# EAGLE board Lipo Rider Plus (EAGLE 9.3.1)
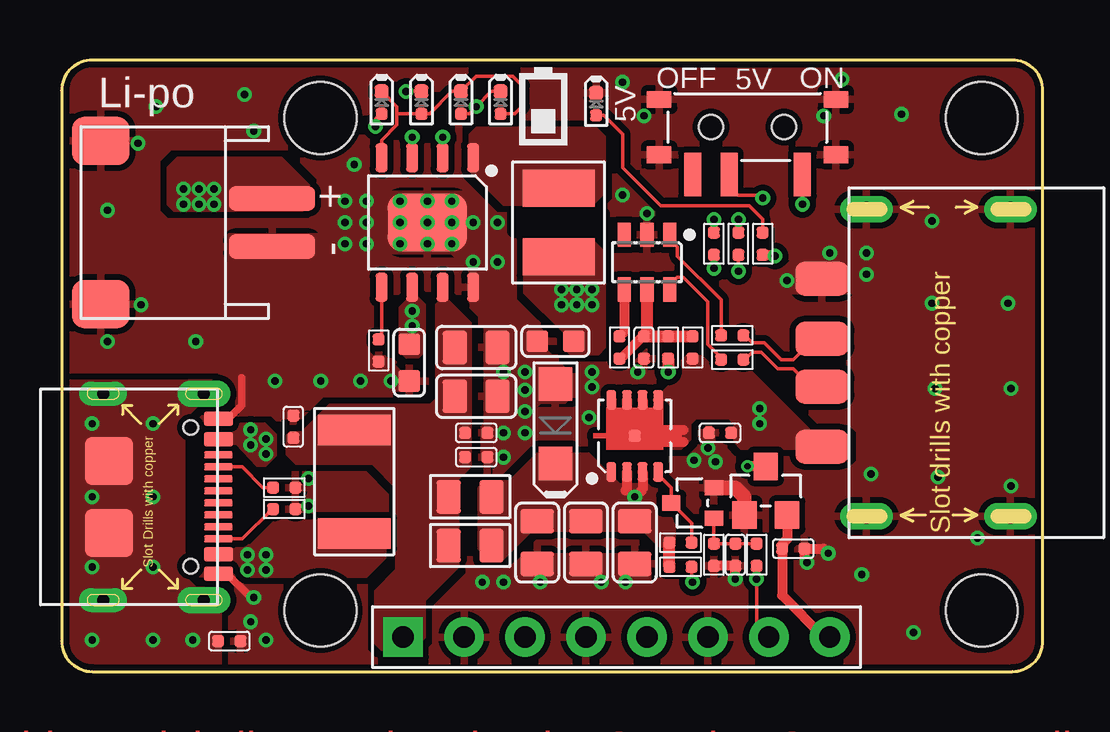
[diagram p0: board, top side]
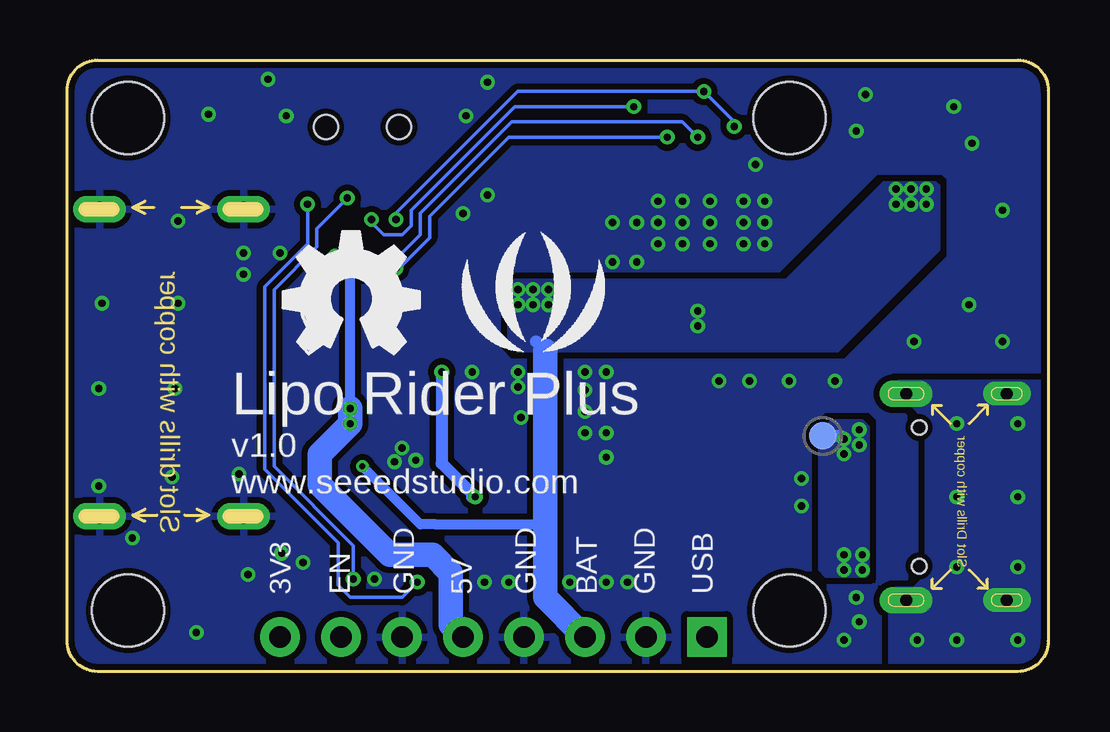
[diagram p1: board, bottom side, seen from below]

Size 40.88 x 25.48 mm. Coordinates in mm from the lower left corner, seen from the top.
Outline: 0,24.21 0,1.27 arc90 1.27,0 39.61,0 arc90 40.88,1.27 40.88,24.21 arc90 39.61,25.48 1.27,25.48 arc90 0,24.21
Copper layers (1*16): Top 0.035mm / dielectric 1.5mm / Bottom 0.035mm
Design rules "SeeedStudio_2layer_DRU_no_angle_20140221 *": minimum track width 1mil, minimum drill 10mil, track to track 6mil, track to pad 6mil, pad to pad 6mil, via to via 6mil, smd to smd 0mil, copper to edge 10mil, drill to drill 10mil, minimum pad ring 4mil, minimum via ring 4mil, stop-mask expansion 2mil, vias tented up to drill 25mil, thermal gap 10mil
Holes 3 mm at 10.78,23.07 10.78,2.54 38.34,23.07 38.34,2.54
tRestrict: area 18.8,18.3 to 22.6,19.1

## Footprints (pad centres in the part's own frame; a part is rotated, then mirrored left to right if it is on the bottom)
C0402 = smd 0.5 x 0.5: 1 -0.463,0; 2 0.463,0
C0603 = smd 0.889 x 0.889: 1 -0.762,0; 2 0.762,0
C0805 = smd 1.016 x 1.397: 1 -0.889,0; 2 0.889,0
ESD-0402 = smd 0.5 x 0.5: 1 -0.463,0; 2 0.463,0
LED-0402 = smd 0.5 x 0.5: + 0.463,0 | smd 0.58 x 0.58: - -0.468,0
SOD-123 = smd 1.397 x 1.397: + 1.651,0; - -1.651,0
F1812 = smd 1.27 x 3.048: 1 -2.159,0; 2 2.159,0
F0805 = smd 1.016 x 1.397: 1 -0.889,0; 2 0.889,0
USB4+4P-2.0-14.6X10.6X5.72MM = smd 1.4 x 2.2: 1 -3.5,0.5; 2 -1,0.5; 3 1,0.5; 4 3.5,0.5 | drill 0.6 pad 1.1 long: S1 -6.4,-1.35; S2 6.4,-1.35; S3 -6.4,-7.35; S4 6.4,-7.35
H8-2.54-C65D35MIL = drill 0.889 pad 1.651 square: 1 0,8.89 | drill 0.889 pad 1.651: 2 0,6.35; 3 0,3.81; 4 0,1.27; 5 0,-1.27; 6 0,-3.81; 7 0,-6.35; 8 0,-8.89
HW2-SMD-2.0-90D = smd 2 x 2.4: 3 3.4,-2.181; 4 -3.4,-2.181 | smd 1 x 3.6: + -1,4.953; - 1,4.953
L4.4X3.0MM = smd 1.55 x 3: 1 -1.425,0; 2 1.425,0
DFN8P-0.65-3X3X0.8MM = smd 0.8 x 0.4: 1 -1.5,0.975; 2 -1.5,0.325; 3 -1.5,-0.325; 4 -1.5,-0.975; 5 1.5,-0.975; 6 1.5,-0.325; 7 1.5,0.325; 8 1.5,0.975 | smd 0.508 x 0.508: 9 0,0
SOT-323 = smd 0.762 x 0.635: 1 0.889,-0.635; 2 0.889,0.635; 3 -0.889,0
R0402 = smd 0.5 x 0.5: 1 -0.463,0; 2 0.463,0
SW7-SMD-L6.7X2.7X3.2MM = smd 1.8 x 0.7: 1 1.978,2.286; 2 1.978,-0.762; 3 1.978,-2.286 | smd 0.7 x 1.016: SS1 -1.15,-3.683; SS2 1.15,-3.683; SS3 1.15,3.683; SS4 -1.15,3.683 | hole 1: 0,-1.524; 0,1.524
TP-D45MIL = smd 1.143 x 1.143: T 0,0
ESOP8L-1.27-5X3.9MM = smd 0.5 x 1.2: 1 -1.905,-2.7; 2 -0.635,-2.7; 3 0.635,-2.7; 4 1.905,-2.7; 5 1.905,2.7; 6 0.635,2.7; 7 -0.635,2.7; 8 -1.905,2.7 | smd 3.3 x 2.4: PAD 0,0
SOT-23-6 = smd 0.55 x 1.016: 1 -0.95,-1.143; 2 0,-1.143; 3 0.95,-1.143; 4 0.95,1.143; 5 0,1.143; 6 -0.95,1.143
SOT-23 = smd 1.016 x 1.143: 1 -0.889,-1.016; 2 0.889,-1.016; 3 0,1.016
USB2.0-TYPE-C = smd 1.2 x 0.6: A1_B12 0.05,3.25; A4_B9 0.05,2.4; B1_A12 0.05,-3.2; B4_A9 0.05,-2.4 | smd 1.2 x 0.3: A5 0.05,1.25; A6 0.05,0.25; A7 0.05,-0.25; A8 0.05,-1.25; B5 0.05,-1.75; B6 0.05,-0.75; B7 0.05,0.75; B8 0.05,1.75 | drill 0.5 pad 1 long: S1 -4.75,4.3; S2 -4.75,-4.3 | drill 0.5 pad 1.1 long: S3 -0.55,4.3; S4 -0.55,-4.3 | smd 2 x 2: S5 -4.5,1.5; S6 -4.5,-1.5 | hole 0.6: -1.1,-2.89; -1.1,2.89

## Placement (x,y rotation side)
C1  100nF  [C0402]  17.27,8.93 0 top
C2  100nF  [C0402]  17.27,9.95 0 top
C3  10uF  [C0603]  14.48,12.87 270 top
C4  10uF  [C0603]  20.57,13.76 180 top
C5  10uF/10V  [C0805]  17.27,11.47 180 top
C6  10uF/10V  [C0805]  17.27,13.5 180 top
C7  10uF/10V  [C0805]  21.84,5.37 90 top
C8  10uF/10V  [C0805]  19.81,5.37 90 top
C9  10uF/10V  [C0805]  23.88,5.37 90 top
C12  100nF  [C0402]  30.48,5.12 0 top
C13  100nF  [C0402]  24.26,13.5 270 top
C42  10nF  [C0402]  28.07,4.87 270 top
C43  100nF  [C0402]  27.43,9.95 180 top
D1  ESDPSA0402V05  [ESD-0402]  9.65,10.2 270 top
D2  GREEN  [LED-0402]  13.34,23.7 270 top
D3  GREEN  [LED-0402]  14.99,23.7 270 top
D4  GREEN  [LED-0402]  18.29,23.7 270 top
D5  GREEN  [LED-0402]  16.64,23.7 270 top
D6  MMSZ4689-E3-08  [SOD-123]  20.57,10.33 90 top
D7  GREEN  [LED-0402]  22.27,23.64 270 top
F1  3A  [F1812]  12.19,7.91 90 top
FB1  1.5A  [F0805]  17.02,5.25 0 top
FB2  1.5A  [F0805]  17.02,7.28 0 top
FR1  SEEEDSTUDIO-OPEN-SCH-FRAME-BIG  [SEEEDSTUDIO-PCB-FRAME]  not placed on the board
FR2  SEEEDSTUDIO-OPEN-SCH-FRAME-BIG  [SEEEDSTUDIO-PCB-FRAME]  not placed on the board
J2  [USB4+4P-2.0-14.6X10.6X5.72MM]  32.18,12.87 90 top
J3  [H8-2.54-C65D35MIL]  23.11,1.44 90 top
J4  320110026  [HW2-SMD-2.0-90D]  3.81,18.71 270 top
L1  1uF  [L4.4X3.0MM]  20.7,18.71 90 top
Q1  AON7403  [DFN8P-0.65-3X3X0.8MM]  23.88,9.82 90 top
Q2  2N7002PW  [SOT-323]  26.29,7.03 0 top
R1  56k  [R0402]  13.21,13.38 90 top
R2  1k  [R0402]  27.18,17.82 90 top
R3  1k  [R0402]  29.21,17.82 270 top
R4  DNP  [R0402]  25.27,13.5 270 top
R5  0R  [R0402]  23.24,13.5 270 top
R6  22R  [R0402]  27.94,12.99 0 top
R7  5.1k  [R0402]  9.27,7.66 180 top
R8  5.1k  [R0402]  9.27,6.77 0 top
R9  1k  [R0402]  28.19,17.82 90 top
R10  22R  [R0402]  27.94,14.01 0 top
R11  2.2k  [R0402]  26.29,13.5 270 top
R12  0R  [C0402]  6.99,1.27 0 top
R32  100k  [R0402]  25.78,5.37 0 top
R46  100k  [R0402]  27.18,4.87 90 top
R47  10k  [R0402]  25.78,4.36 180 top
R48  1k  [R0402]  28.96,4.87 90 top
SW1  311030001  [SW7-SMD-L6.7X2.7X3.2MM]  28.57,22.69 270 top
TP1  TEST  [TP-D45MIL]  9.4,9.82 0 bottom
U1  ETA9740  [ESOP8L-1.27-5X3.9MM]  15.24,18.71 180 top
U2  [SOT-23-6]  24.38,17.06 180 top
U3  [SOT-23]  29.34,7.53 0 top
U$1  [SEEED-SILK-TNAME-280*268MIL]  21.46,15.03 0 bottom
U$2  [OSHW_FILLX200_NOTEXT_TNAME]  31.88,13.25 0 bottom
USB2  TYPE-C  [USB2.0-TYPE-C]  6.48,7.28 0 top

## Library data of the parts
C1-C9 C12 C13 C42 C43 D1-D7 F1 FB1 FB2 L1 Q1 Q2 R1-R12 R32 R46-R48 SW1 = Discrete-new
FR1 FR2 = moudle-new
J2-J4 USB2 = Connector-new
TP1 = Discrete-new; PARTNO: DNP
U1-U3 = IC-new
U$1 U$2 = logo

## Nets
3V3: C12.1 J3.8 U3.2
5V: C43.1 J2.1 J3.5 Q1.5 Q1.6 Q1.7 Q1.8 Q1.9 R3.2 R11.2
BAT: C3.1 C4.1 J3.3 J4.+ L1.1 U1.6 U3.3
D+: J2.3 R10.2
D-: J2.2 R6.2
EN: J3.7 R48.1 SW1.2
GND: C1.2 C2.2 C3.2 C4.2 C5.1 C6.1 C7.1 C8.1 C9.1 C12.2 C13.2 C42.2 C43.2 D1.1 D6.+ D7.- J2.4 J2.S1 J2.S2 J2.S3 J2.S4 J3.2 J3.4 J3.6 J4.3 J4.4 J4.- Q2.2 R1.1 R7.1 R8.2 R12.2 R46.1 SW1.SS1 SW1.SS2 SW1.SS3 SW1.SS4 U1.8 U1.PAD U2.2 U3.1 USB2.A1_B12 USB2.B1_A12
LED1: D2.+ D3.- R2.2
LED2: D4.- D5.+ R9.2
LED3: D2.- D3.+ D4.+ D5.- U1.4
N$1: R7.2 USB2.A5
N$2: R8.1 USB2.B5
N$3: R47.1 SW1.1
N$4: F1.1 TP1.T USB2.A4_B9 USB2.B4_A9
N$6: D7.+ R3.1
N$7: R1.2 U1.5
N$8: L1.2 U1.1
N$9: R9.1 U1.3
N$10: R5.1 U2.4
N$11: C13.1 R4.1 R5.2 R11.1 U2.5
N$12: R2.1 U1.2
N$13: R6.1 U2.6
N$14: R10.1 U2.1
N$49: Q1.4 Q2.3 R32.2
N$52: C42.1 Q2.1 R46.2 R48.2
SHIELD: R12.1 USB2.S1 USB2.S2 USB2.S3 USB2.S4 USB2.S5 USB2.S6
VCC_5V: C7.2 C8.2 C9.2 D6.- FB1.2 FB2.2 Q1.1 Q1.2 Q1.3 R4.2 R32.1 R47.2
VUSB: C1.1 C2.1 C5.2 C6.2 D1.2 F1.2 FB1.1 FB2.1 J3.1 U1.7

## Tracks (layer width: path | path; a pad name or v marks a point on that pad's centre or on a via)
3V3
  Top 0.406: J3.8 31.75,1.44 30.02,3.17 C12.1 30.02,5.29 30.23,5.5 U3.2
5V  (via drill 0.3 pad 0.61)
  Top 0.406: 29.04,11.01 v29.08,10.96 | R3.2 29.67,17.36 v29.72,17.31 | Q1.5 24.85,10.54 24.77,10.45 | Q1.6 24.2,10.64 24.77,10.07 24.89,10.07 | Q1.7 23.55,10.4 23.62,10.33 | Q1.8 22.9,10.41 22.99,10.33 | 24.89,10.07 25.91,10.07 | 24.89,10.07 24.89,9.69 25.02,9.56 25.65,9.56 | 25.65,9.56 25.91,9.56 | 25.65,9.56 25.65,9.95
  Bottom 0.406: v29.08,10.96 29.08,16.68 v29.72,17.31
  Bottom 1.016: v29.08,10.96 v29.08,10.33 30.35,9.06 30.35,7.79 27.43,4.87 25.65,4.87 24.89,4.1 24.89,1.95 J3.5
  pour Top (isolate 0.254, no thermals): 32.51,8.8 31.37,8.8 30.86,9.31 28.32,9.31 28.07,9.56 28.07,10.33 27.81,10.58 26.42,10.58 26.16,10.33 26.16,9.67 25.8,9.31 23.11,9.31 22.73,9.69 22.73,10.58 22.99,10.84 24.64,10.84 24.89,11.09 24.89,11.47 25.78,12.36 25.78,12.87 26.04,13.12 26.67,13.12 27.3,12.49 28.7,12.49 31.24,9.95 32.51,9.95 32.77,9.69 32.77,9.06
BAT  (via drill 0.25 pad 0.51, 0.3 pad 0.61)
  Top 0.406: U3.3 v28.57,8.55
  Bottom 0.406: 20.95,6.26 21.08,6.14 25.27,6.14 25.53,6.14 26.16,6.14 v28.57,8.55
  Bottom 0.508: 20.95,13.38 C4.1
  Bottom 1.016: 20.95,13.38 20.95,6.26 20.95,3.09 J3.3
  other vias: 22.1,15.28 21.46,15.28 21.46,15.91 22.1,15.91 20.83,15.91 20.83,15.28 6.35,20.11 6.35,19.47 5.71,19.47 5.71,20.11 5.08,20.11 5.08,19.47 14.61,15.03 14.61,14.39
  pour Top (isolate 0.254, no thermals): 10.03,19.22 4.7,19.22 4.45,19.47 4.45,21 4.83,21.38 9.14,21.38 10.29,20.23 10.29,19.47
  pour Top (isolate 0.254, no thermals): 14.61,16.3 14.48,16.17 14.48,15.53 14.1,15.15 14.1,13.38 14.35,13.12 14.86,13.12 15.11,13.38 15.11,15.28 14.86,15.53 14.73,15.66 14.73,16.17
  pour Top (isolate 0.254, no thermals): 22.1,13.25 21.21,13.25 20.95,13.5 20.95,14.14 19.3,15.79 19.3,17.69 19.56,17.95 22.1,17.95 22.61,17.44 22.61,13.5 22.35,13.25
  pour Bottom (isolate 0.254, no thermals): 21.84,16.3 10.92,16.3 6.86,20.36 4.7,20.36 4.57,20.23 4.57,17.57 8.76,13.38 22.1,13.38 22.48,13.76 22.48,16.04 22.23,16.3
D+
  Top 0.152: R10.2 28.45,14.01 28.77,13.69 29.27,13.69 29.97,12.99 30.48,12.99 31.35,13.87 J2.3
D-
  Top 0.152: R6.2 28.45,12.99 28.77,13.31 29.15,13.31 29.84,12.61 30.48,12.61 31.18,11.91 31.23,11.87 J2.2
EN  (via drill 0.3 pad 0.61)
  Top 0.152: 28.96,4.49 R48.1 v28.96,3.85 28.96,1.95 J3.7 | v29.21,19.73 29.08,19.85 28.19,19.85 27.81,20.23 SW1.2
  Bottom 0.152: v28.96,3.85 28.96,5.25 32.26,8.55 32.26,15.91 30.48,17.69 30.48,18.45 v29.21,19.73
GND  (via drill 0.3 pad 0.61)
  Top 0.305: USB2.B1_A12 6.88,4.08 7.75,3.21 | USB2.A1_B12 6.93,10.53 7.49,11.09 7.49,12.23
  Top 0.406: R46.1 C42.2 v28.07,3.85 | v31.05,4.55 30.94,4.66 C12.2 31.75,5.12 v31.94,4.93
  Top 0.61: Q2.2 28.07,7.66 28.45,7.28 U3.1
  other vias: 18.41,9.95 18.41,8.93 19.3,9.95 19.3,10.84 19.3,11.72 19.3,12.49 18.41,12.49 15.24,18.71 15.24,19.6 15.24,17.82 14.1,17.82 14.1,18.71 14.1,19.6 16.26,19.6 16.26,18.71 16.26,17.82 17.14,17.06 18.16,17.06 18.16,18.71 17.14,18.71 12.7,19.6 12.7,18.71 12.7,17.82 11.81,17.82 11.81,18.71 11.81,19.6 13.72,12.11 12.45,12.11 10.79,12.11 8.89,12.11 3.3,15.28 3.17,22.01 19.94,3.72 18.41,3.72 17.53,3.72 22.48,3.72 23.5,3.72 24,12.49 26.92,9.31 26.35,8.8 27.24,8.74 24.38,19.09 23.37,24.55 24.26,23.15 32.51,24.68 31.75,23.15 8,3.09 7.87,2.07 8.51,1.31 3.94,23.54 7.62,24.04 1.91,19.22 5.59,13.76 22.1,12.49 32,17.44 33.53,17.44 33.53,16.55 30.23,16.3 23.37,19.85 22.1,11.85 21.97,10.58 1.91,13.76 8,22.52 12.19,21.12 10.29,8.04 10.29,6.9 33.72,8.23 33.34,4.04 38.16,5.56 39.56,7.72 36.51,8.1 36.39,11.79 39.56,11.79 39.43,15.34 36.26,15.34 36.26,18.77 34.99,23.22 35.5,1.63
  pour Top (isolate 0.254, no thermals): 17.65,8.68 18.41,8.68 19.56,9.82 19.56,10.84 19.94,11.22 20.95,11.22 21.21,11.47 22.23,11.47 22.35,11.6 22.35,12.11 22.1,12.36 21.21,12.36 20.19,13.38 20.19,14.01 18.54,15.66 18.54,18.71 18.29,18.96 17.91,18.96 16.89,19.98 11.81,19.98 11.56,19.73 11.56,18.96 10.79,18.2 6.99,18.2 6.99,13.38 8.64,11.72 8.64,10.96 9.02,10.58 9.78,10.58 10.92,11.72 14.48,11.72 14.73,11.98 14.73,12.36 14.61,12.49 14.1,12.49 13.46,13.12 12.97,13.12 12.67,13.42 12.67,16.77 13.34,17.44 16.26,17.44 17.02,16.68 17.02,15.41 17.65,14.77 17.65,10.33 17.53,10.2 17.53,8.8
  pour Top (isolate 0.254, no thermals): 23.75,4.87 24.13,4.87 24.51,4.49 24.51,3.34 24.13,2.96 16.76,2.96 16.51,3.21 16.51,3.6 17.02,4.1 18.54,4.1 19.3,4.87
  pour Top (isolate 0.254, no thermals): 26.8,10.07 26.67,9.95 26.67,9.44 26.16,8.93 26.16,8.55 26.29,8.42 26.42,8.42 26.8,8.04 26.8,7.53 26.92,7.41 27.94,7.41 28.26,7.72 28.26,8.04 27.81,8.8 27.18,9.56 27.18,9.95 27.05,10.07
  pour Top (isolate 0.254, no thermals): 8.38,3.47 8.13,3.47 7.37,2.71 7.37,1.18 7.62,0.93 8.64,0.93 8.89,1.18 8.89,3.09 8.51,3.47
  pour Top (isolate 0.254, no thermals): 32.51,15.79 33.91,15.79 34.29,16.17 34.29,17.44 34.04,17.69 30.99,17.69 29.97,16.68 29.97,16.17 30.23,15.91 30.35,15.79
  pour Top (isolate 0.254, rank 6): -0.64,26.07 41.7,26.07 41.7,-0.59 -0.64,-0.59
  pour Bottom (isolate 0.254, rank 6): -0.64,26.07 41.7,26.07 41.7,-0.59 1.91,-0.59 1.91,-1.23 -0.64,-1.23
  pour Top (isolate 0.254): 31.62,5.63 31.24,5.63 30.73,5.12 30.73,3.47 30.99,3.21 31.24,3.21 31.5,3.47 31.5,3.98 32.13,4.61 32.13,5.25 31.75,5.63
LED1  (via drill 0.3 pad 0.61)
  Top 0.152: D2.+ 13.29,23.24 13.08,23.03 v13.08,22.71 | R2.2 v27.18,18.84 | D3.- v14.35,24.17
  Bottom 0.152: v27.18,18.84 27.18,19.09 22.1,24.17 v14.35,24.17 13.08,22.9 v13.08,22.71
LED2  (via drill 0.3 pad 0.61)
  Top 0.152: R9.2 v28.19,18.84 | D4.- 17.91,24.17 v17.27,23.54 16.98,23.24 D5.+
  Bottom 0.152: v17.27,23.54 22.23,23.54 26.54,19.22 26.54,18.58 26.92,18.2 27.69,18.2 28.19,18.71 v28.19,18.84
LED3
  Top 0.152: U1.4 13.34,22.14 13.97,22.77 13.97,23.28 | 13.97,23.28 13.97,23.54 D2.- | D2.- | 13.97,23.28 14.01,23.24 D3.+ 15.32,23.24 16.26,24.17 D5.- 17.27,24.8 18.8,24.8 19.18,24.42 19.18,23.54 18.88,23.24 D4.+
N$1
  Top 0.152: USB2.A5 7.51,8.53 8.38,7.66 R7.2
N$2
  Top 0.152: USB2.B5 7.52,5.53 8.76,6.77 R8.1
N$3  (via drill 0.3 pad 0.61)
  Top 0.152: R47.1 26.24,3.77 v26.29,3.72 | SW1.1 v30.86,19.47
  Bottom 0.152: v26.29,3.72 26.92,3.09 29.08,3.09 29.59,3.6 29.59,5.37 32.64,8.42 32.64,16.04 30.86,17.82 v30.86,19.47
N$4  (via drill 0.3 pad 0.61)
  Bottom 0.508: TP1.T 8.64,9.82 v8.51,9.69
  other vias: 8.51,9.06 7.87,9.44 7.87,10.07 7.75,4.87 8.51,4.87 8.51,4.23 7.75,4.23
  pour Top (isolate 0.254, no thermals): 6.16,9.82 6.99,9.82 7.47,10.3 8.45,10.3 8.89,9.86 8.89,9.01 8.48,8.59 8.15,8.59 7.3,9.5 6.22,9.5 6.1,9.63 6.1,9.76
  pour Bottom (isolate 0.254, no thermals): 7.87,10.45 7.75,10.45 7.49,10.2 7.49,4.1 7.62,3.98 9.27,3.98 9.53,4.23 9.53,9.95 9.02,10.45
  pour Top (isolate 0.254, no thermals): 6.35,4.99 7.11,4.99 7.37,5.25 7.87,5.25 8.89,6.26 13.21,6.26 13.46,6.01 13.46,4.74 12.7,3.98 7.87,3.98 7.11,4.74 6.35,4.74 6.22,4.87
N$6
  Top 0.152: R3.1 29.21,18.84 28.64,19.41 24.96,19.41 23.37,21 23.37,22.39 22.58,23.18 D7.+
N$7
  Top 0.152: U1.5 13.34,13.96 R1.2
N$8
  pour Top (isolate 0.254, no thermals): 17.02,20.87 17.02,22.36 17.3,22.65 22.25,22.65 22.61,22.29 22.61,19.98 22.1,19.47 18.41,19.47
N$9  (via drill 0.3 pad 0.61)
  Top 0.152: U1.3 v14.61,22.27 | v28.19,16.68 R9.1
  Bottom 0.152: v28.19,16.68 27.43,17.44 26.92,17.44 26.16,18.2 26.16,19.09 22.35,22.9 15.24,22.9 v14.61,22.27
N$10
  Top 0.406: U2.4 23.43,14.16 R5.1
N$11
  Top 0.406: R5.2 23.29,13.04 24.21,13.96 C13.1
  Top 0.508: U2.5 24.38,14.14 24.26,14.01 C13.1 R4.1 R11.1
N$12  (via drill 0.3 pad 0.61)
  Top 0.152: U1.2 v15.88,22.27 | R2.1 v27.18,16.8
  Bottom 0.152: v15.88,22.27 22.48,22.27 25.78,18.96 25.78,18.07 27.05,16.8 v27.18,16.8
N$13
  Top 0.152: R6.1 27.48,13.07 26.92,13.63 26.92,15.41 25.91,16.42 25.65,16.42 25.33,16.1 U2.6
N$14
  Top 0.152: R10.1 27.48,15.49 25.65,17.31 25.65,17.69 25.33,18.01 U2.1
N$49
  Top 0.152: R32.2 26.24,6.18 Q2.3 25.4,7.66 24.85,8.21 Q1.4
N$52
  Top 0.152: R48.2 C42.1 R46.2 Q2.1
SHIELD  (via drill 0.3 pad 0.61)
  other vias: 5.46,1.31 3.81,1.31 1.27,1.31 1.27,4.36 3.81,4.36 3.81,7.28 1.27,7.28 1.27,10.33 3.81,10.33
  pour Top (isolate 0.254, no thermals): 0,12.11 6.22,12.11 6.48,11.85 6.48,11.47 6.22,11.22 5.76,11.22 5.08,10.53 5.08,3.98 5.59,3.47 6.35,3.47 6.6,3.21 6.6,0.04 0,0.04
  pour Bottom (isolate 0.254, no thermals): 0,12.11 6.22,12.11 6.48,11.85 6.48,11.47 6.22,11.22 5.82,11.22 5.08,10.48 5.08,3.99 5.6,3.47 6.35,3.47 6.6,3.21 6.6,0.04 0,0.04
VCC_5V  (via drill 0.3 pad 0.61)
  Top 0.406: Q1.2 23.55,7.59 23.5,7.53 | Q1.3 24.2,7.6 v23.88,7.28
  Top 0.508: R4.2 v25.27,12.49 | R47.2 R32.1
  Bottom 0.508: v25.27,12.49 25.27,8.68 v23.88,7.28 24,7.28
  pour Top (isolate 0.254, no thermals): 17.65,7.91 18.67,7.91 19.81,9.06 21.97,9.06 23.24,7.79 24.64,7.79 25.15,7.03 25.53,6.01 25.53,5.37 25.4,5.25 24.89,5.25 24.26,5.88 19.56,5.88 18.41,4.74 17.78,4.74 17.4,5.12 17.4,7.66
VUSB
  pour Top (isolate 0.254, no thermals): 15.88,16.17 15.75,16.04 15.75,15.41 15.62,15.28 15.62,11.34 15.37,11.09 11.18,11.09 10.03,9.95 9.53,9.95 9.4,9.82 9.4,9.06 9.78,8.68 12.95,8.68 13.97,7.66 13.97,4.23 13.08,3.34 13.08,1.18 13.34,0.93 14.61,0.93 15.11,1.44 15.11,2.96 16.51,4.36 16.51,8.04 17.02,8.55 17.02,14.52 16,15.53 16,16.04

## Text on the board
tNames: OFF | 5V | ON | Li-po | 5V | + | -
bNames: Lipo Rider Plus | v1.0 | www.seeedstudio.com | USB | GND | BAT | GND | 5V | GND | EN | 3V3

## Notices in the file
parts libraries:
moudle-new: This work is licensed under the Creative Commons Attribution 4.0 International License.
To view a copy of this license,visit:
http://creativecommons.org/licenses/by-sa/4.0
